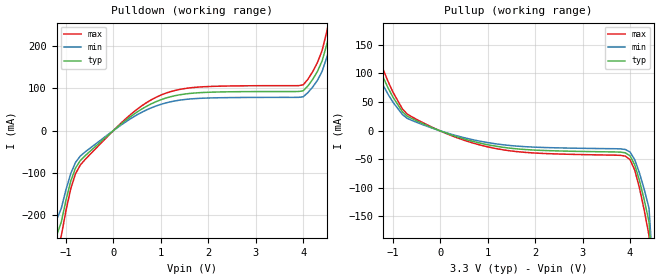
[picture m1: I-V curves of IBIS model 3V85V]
[IBIS Ver]   2.1
[File name]   ics501_3.ibs
[File Rev]   2.0
[Date]   6/2/00
[Source]   ICS MicroClock Applications Engineering 2
[Disclaimer] This information is for modeling purposes only, and is
(C) Copyright Integrated Circuit Systems, Inc. 1997-2001
   All rights reserved
ICS hereby grants the user of this IBIS model a non-exclusive,
nontransferable license to use this IBIS model under the following terms.
Before using this IBIS model, the user should read this license.
If the user does not accept these terms,  the IBIS model should be
returned to ICS within 30 days.
   The user is granted this license only to use the IBIS model and
is not granted rights to sell, load, rent, lease or license the IBIS
model in whole or in part, or in modified form to anyone other than
user. User may modify the IBIS model to suit its specific
applications but rights to derivative works and such modifications
shall belong to ICS.
   This IBIS model is provided on an "AS IS" basis and ICS makes
absolutely no warranty with respect to the information contained
herein. ICS DISCLAIMS AND CUSTOMER WAIVES ALL WARRANTIES, EXPRESS
OR IMPLIED, INCLUDING WARRANTIES OF MERCHANTABILITY OR FITNESS FOR
A PARTICULAR PURPOSE. The entire risk as to quality and performance
is with the Customer. ACCORDINGLY, IN NO EVENT SHALL THE COMPANY BE
LIABLE FOR ANY DAMAGES, WHETHER IN CONTRACT OR TORT,INCLUDING ANY
LOST PROFITS OR OTHER INCIDENTAL, CONSEQUENTIAL, EXEMPLARY, OR
PUNITIVE DAMAGES ARISING OUT OF THE USE OR APPLICATION OF THE IBIS
model provided in this package. Further, ICS reserves the right to
make changes without notice to any product herein to improve
reliability, function, or design. ICS does not convey any license
under patent rights or any other intellectual property rights,
including those of third parties.
   ICS is not obligated to provide maintenance or support
for the licensed IBIS model.
[Component]   ICS501
[Manufacturer] Integrated Circuit Systems Inc.
[Package]
|   typ   min   max
R_pkg   40m   35m   45m
L_pkg   1.65nH   1.35nH   1.95nH
C_pkg   0.24pF   0.14pF   0.34pF
[pin]   signal_name   model_name   R_pin   L_pin   C_pin
   5   CLK   3V85V
| Models and submodels in the file (1): 3V85V (Output)
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|   ICS501 3.3V Clock Drive Model
| This model is suitable for CLK output pins on the
| ICS501
[Model]   3V85V
Model_type   Output
Polarity   Non-Inverting
|   typ   min   max
C_comp   5pF   4pF   6pF
|   typ   min   max
[Voltage range]  3.3V   3.15V   3.45V
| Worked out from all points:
|   slope of the pulldown table from 0 to 0.495 V, typ, clamps not added: 11.3 ohm
|   slope of the pullup table from 0 to 0.495 V, typ, clamps not added: 35.6 ohm
[pulldown]
|Voltage I (typ)   I (min)   I (max)
-3.3V     -3A        -3A        -3A
-1.2V     -250.1mA   -212.6mA   -287.6mA
-1.1V     -218mA     -185.3mA   -250.8mA
-900mV    -120.3mA   -102.2mA   -138.3mA
-700mV    -71.62mA   -60.87mA   -82.36mA
300mV     27.87mA    23.69mA    32.06mA
1V        73.25mA    62.26mA    84.24mA
4V        94.35mA    80.2mA     108.5mA
4.3V      140.2mA    119.2mA    161.3mA
4.5V      205.6mA    174.7mA    236.4mA
4.6V      250.2mA    212.7mA    287.7mA
6.6V      3A         3A         3A
[pullup]
|Voltage I (typ)   I (min)   I (max)
-3.3V     3A         3A         3A
-1.4V     161.3mA    137.1mA    185.5mA
-1.2V     92.17mA    78.34mA    106mA
-800mV    32.95mA    28mA       37.89mA
-200mV    5.955mA    5.062mA    6.848mA
1.4V      -30.19mA   -25.66mA   -34.72mA
3.9V      -39.01mA   -33.16mA   -44.86mA
4V        -44.29mA   -37.65mA   -50.93mA
4.1V      -60.33mA   -51.28mA   -69.37mA
4.2V      -87.91mA   -74.72mA   -101.1mA
4.4V      -159.9mA   -135.9mA   -183.9mA
6.6V      -3A        -3A        -3A
[Ramp]
|   typ   min   max
dV/dt_r   1.01/0.94n   0.96/1.04n   1.06/0.85n
dV/dt_f   1.62/0.53n   1.54/0.58n   1.70/0.48n
